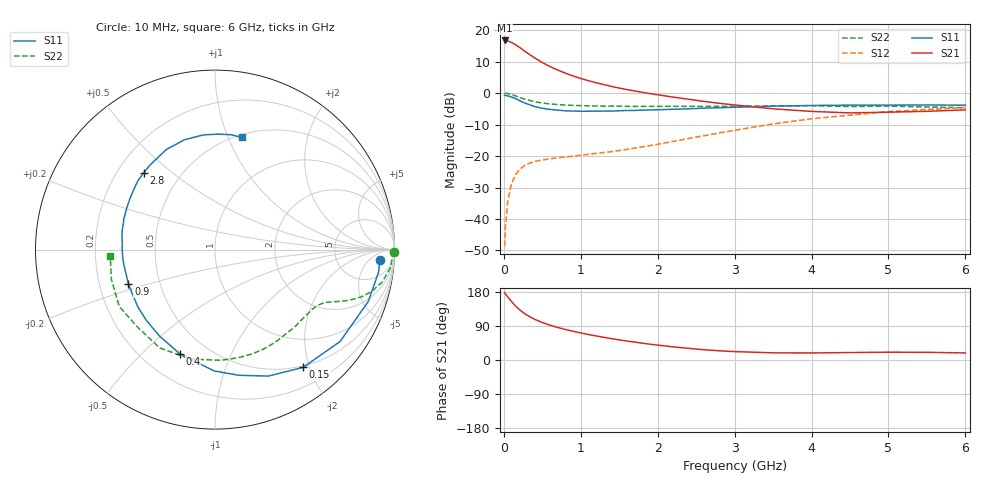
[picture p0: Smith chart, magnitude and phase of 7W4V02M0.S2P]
! Infineon Technologies  Discrete & RF Semiconductors
! BFS17W
! Si NPN RF Bipolar Junction Transistor in SOT323
! VCE = 4 V  IC = 2 mA
! Common Emitter S-Parameters:  August  1999
# GHz  S  MA  R  50
!  f  S11  S21  S12  S22
! GHz  MAG  ANG  MAG  ANG  MAG  ANG  MAG  ANG
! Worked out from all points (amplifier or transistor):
!   36 points, 10 MHz to 6 GHz, reference 50 ohm
!   highest |S21| = 16.7 dB at 10 MHz (marker M1)
!   |S21| within 3 dB of that: start of sweep to 248.4 MHz
!   unconditionally stable (mu >= 1): 825.8 MHz to 3.277 GHz; 4.01 GHz to end of sweep
!   at 250 MHz: K = 0.36, MSG = 18.5 dB, |S12| = -23.4 dB
!   at 1.4 GHz: K = 1.30, MAG = 7.1 dB, |S12| = -18.6 dB
!   at 6 GHz: K = 1.09, MAG = -2.2 dB, |S12| = -4.6 dB
!   S11 on the Smith chart (normalised r, x): 10 MHz: 15, -11; 150 MHz: 0.48, -1.90; 400 MHz: 0.35, -0.66; 900 MHz: 0.33, -0.17; 2.8 GHz: 0.31, +0.40; 6 GHz: 0.53, +1.12
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0.01  0.9196 -3.6  6.845 178.0  0.0037 85.3  0.9994 -0.7
0.02  0.9204 -7.7  6.835 174.7  0.0072 87.4  0.989 -2.3
0.05  0.9016 -18.7  6.731 166.5  0.019 80.5  0.9833 -5.8
0.1  0.8649 -36.3  6.363 154.3  0.0365 70.6  0.95 -10.9
0.15  0.8195 -53.2  5.873 142.9  0.0497 62.1  0.9034 -15.0
0.2  0.765 -67.1  5.364 133.4  0.0603 56.3  0.8586 -17.8
0.25  0.7127 -79.3  4.83 125.4  0.0677 51.3  0.8149 -19.9
0.3  0.6758 -90.5  4.367 118.6  0.0743 47.7  0.7821 -21.4
0.4  0.6125 -108.7  3.619 107.3  0.0816 43.1  0.7282 -23.5
0.5  0.5723 -122.7  3.054 98.9  0.0865 40.8  0.6952 -24.9
0.6  0.5492 -134.3  2.633 91.8  0.0905 39.9  0.6717 -26.3
0.7  0.5349 -143.6  2.32 85.9  0.094 40.5  0.6566 -27.9
0.9  0.5189 -158.5  1.867 75.8  0.0994 41.8  0.6363 -31.4
1.1  0.5146 -170.5  1.571 67.1  0.1065 44.9  0.6264 -35.6
1.4  0.5175 176.0  1.273 56.4  0.1175 50.3  0.6197 -42.5
1.6  0.5285 167.9  1.134 50.0  0.1272 53.8  0.6143 -47.6
2.2  0.5521 149.3  0.862 34.7  0.1705 62.4  0.6163 -63.8
2.8  0.5845 132.8  0.688 24.3  0.2323 64.9  0.6157 -81.5
3.5  0.6203 115.9  0.562 18.9  0.3234 62.0  0.625 -102.5
4.5  0.6422 96.0  0.484 19.7  0.4462 50.2  0.6105 -135.1
5.5  0.6462 81.9  0.513 20.3  0.5489 37.2  0.6007 -163.9
6  0.6422 76.6  0.54 18.6  0.5887 30.9  0.5847 -176.7
